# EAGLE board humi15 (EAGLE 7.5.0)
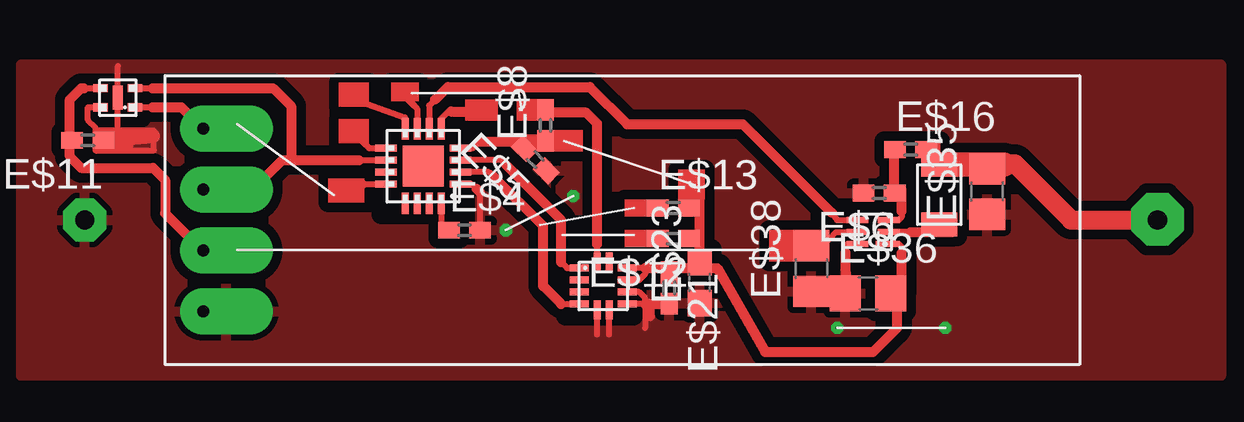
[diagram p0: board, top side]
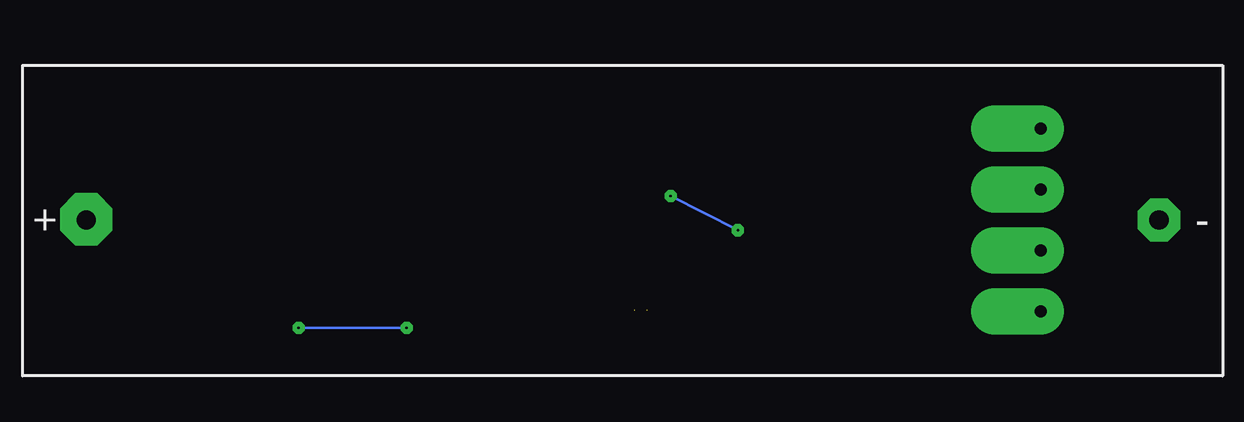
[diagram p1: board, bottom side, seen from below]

No outline drawn. Coordinates in mm, seen from the top.
Copper layers (1*16): Top 0.035mm / dielectric 1.5mm / Bottom 0.035mm
Design rules "default": minimum track width 10mil, minimum drill 24mil, track to track 8mil, track to pad 8mil, pad to pad 8mil, via to via 8mil, smd to smd 8mil, copper to edge 40mil, drill to drill 8mil, minimum pad ring 10mil, minimum via ring 8mil, stop-mask expansion 4mil, vias tented up to drill 0mil, thermal gap 10mil
tRestrict: area 22.7,2.5 to 25.5,5; area 15,6.7 to 18.5,10.5; area 3.1,10.8 to 5,12.2; area 34,4.8 to 36.9,7

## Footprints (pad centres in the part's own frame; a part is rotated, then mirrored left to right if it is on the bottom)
AAA_BATT = drill 0.8 pad 1.778 octagon: P$1 22.35,0; P$2 -22.35,0
OLED_128X32 = drill 0.5 pad 1.93 offset: 1 3.81,-1.587; 2 1.27,-1.587; 3 -1.27,-1.587; 4 -3.81,-1.587
QFN3X3_16 = smd 0.9 x 0.28: 1 -1.8,1; 2 -1.8,0.5; 3 -1.8,0; 4 -1.8,-0.5; 9 1.3,-0.5; 10 1.3,0; 11 1.3,0.5; 12 1.3,1 | smd 0.28 x 0.9: 5 -1,-1.3; 6 -0.5,-1.3; 7 0,-1.3; 8 0.5,-1.3; 13 0.5,1.8; 14 0,1.8; 15 -0.5,1.8; 16 -1,1.8 | smd 1.7 x 1.7: EP -0.25,0.25
C0402 = smd 0.9 x 0.7: 1 -0.65,0; 2 0.65,0
LGA12 = smd 0.8 x 0.3: 1 -0.75,0.5; 2 -0.75,0; 3 -0.75,-0.5; 4 -0.75,-1; 7 1.25,-1; 8 1.25,-0.5; 9 1.25,0; 10 1.25,0.5 | smd 0.3 x 0.8: 5 0,-1.25; 6 0.5,-1.25; 11 0.5,0.75; 12 0,0.75
DSE = smd 0.25 x 1: 1 -0.5,-0.6 | smd 0.25 x 0.9: 2 0,-0.65; 3 0.5,-0.65; 4 0.5,0.65; 5 0,0.65; 6 -0.5,0.65
SH4X = smd 0.6 x 0.35: 1 -0.725,0.4; 2 -0.725,-0.4; 3 0.725,-0.4; 4 0.725,0.4 | smd 0.4 x 1: EP 0,0
C0603 = smd 1.1 x 1: 1 -0.85,0; 2 0.85,0
C0805 = smd 1.3 x 1.5: 1 -0.95,0; 2 0.95,0
L1008 = smd 1 x 1.5: P$1 -1.25,0; P$2 1.25,0

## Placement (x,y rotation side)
E$1  [AAA_BATT]  25,6.5 180 bottom
E$2  [OLED_128X32]  6,6.5 90 top
E$3  [QFN3X3_16]  16.5,9 180 top
E$4  [C0402]  18.48,6.08 0 top
E$5  [C0402]  21.43,9.02 135 top
E$6  [C0402]  35.75,7.62 180 top
E$7  [LGA12]  24,4 0 top
E$8  [C0402]  21.85,10.45 90 top
E$9  [DSE]  35.5,6 90 top
E$10  [SH4X]  4.03,11.6 180 top
E$11  [C0402]  2.77,9.82 180 top
E$12  [C0402]  27.18,5.72 180 top
E$13  [C0402]  27.18,7 0 top
E$16  [C0402]  37.06,9.44 0 top
E$21  [C0402]  27,3.67 270 top
E$23  [C0603]  28.28,3.89 90 top
E$35  [C0805]  40.25,7.69 90 top
E$36  [C0805]  35.29,3.44 0 top
E$38  [C0805]  32.92,4.47 90 top
E$47  [L1008]  38.25,7.56 90 top

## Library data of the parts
E$1 = sb
E$2 = display-lcd
E$3 = renesas
E$4-E$6 E$8 E$11-E$13 E$16 E$21 E$23 E$35 E$36 E$38 = ref-packages
E$7 = st-microelectronics
E$9 = texas
E$10 = sensor
E$47 = rcl

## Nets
GND: E$1.P$2 E$2.4 E$4.2 E$5.1 E$6.2 E$7.5 E$7.6 E$11.1 E$21.2 E$23.1 E$35.1 E$36.1 E$38.1

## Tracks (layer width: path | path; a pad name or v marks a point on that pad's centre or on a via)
GND  (via drill 0.1 pad 0.3)  (2 unrouted)
  Top 0.254: 3.33,11.2 2.77,11.2 2.77,10.68 3.1,10.35 3.1,10.22 4.03,10.22 | 4.03,10.22 4.03,12.93 | 4.03,10.22 5.53,10.22 5.53,9.4 3.1,9.4 3.1,9.93 | 24.5,1.72 E$7.6 | 24,1.72 E$7.5 | 25.5,3.5 25.75,3.5 26,3.25 26,3 | 26,3 25.5,3 | 26,3 26,2 | 34.48,5.5 34.41,5.5 34.35,5.44 34.35,5.14 | 18.5,8 18.77,8 18.98,7.8 | E$4.2 19.12,7.65
  Top 0.406: 26.2,3 26,3 | 26.2,3 27,3 | 26.2,2.5 26.2,3 | 34.38,3.56 34.35,5.14 | 19.12,7.65 18.98,7.8
  Top 0.61: E$11.1 5.47,10 | 32.88,3.56 34.38,3.56 | 4.38,9.62 3.38,9.62
  Bottom 0.1: v34,2 v38.5,2 | v20.2,6.08 v23,7.5
  pour Top (isolate 0.406): 0,0 0,13 50,13 50,0
IRQ
  Top 0.254: 24,5 24,5.5
  Top 0.406: 22.05,10.97 23.55,10.97 24,10.53 24,5.5
PWR
  Top 0.254: 25.5,4 25.75,4 26,4.25 26,4.5 25.5,4.5
  Top 0.406: 36.5,3 36.5,2 35.5,1 31,1 29,4.5 26,4.5
S$1
  Top 0.406: 28.27,4.95 28.27,7.95
S$2
  Top 0.254: 14.2,8 15,8
  Top 0.406: 13.1,8 14.2,8
S$3
  Top 0.254: 17.5,7 17.5,6
S$4
  Top 0.254: 14.35,9.65 14.5,9.5 15,9.5
  Top 0.3: 14.35,9.65 14,10 13.47,10
S$5
  Top 0.254: 14.07,9 15,9
  Top 0.406: 14.07,9 10.88,9 9.38,7.5
S$6
  Top 0.254: 18.8,9.53 18.77,9.5 18.52,9.5
  Top 0.305: 18.8,9.53 19.07,9.78
  Top 0.406: 19.07,9.78 20.62,9.78
  Top 0.61: 20.62,9.78 21.8,9.78
S$7
  Top 0.254: 17.5,10.5 17.5,10.72 17.8,11.03 17.9,11.03 | 18.98,11.03 19.07,11.03
  Top 0.406: 17.9,11.03 18.98,11.03
S$9
  Top 0.254: 16,10.5 16,10.78 14.38,11.35
S$10
  Top 0.8: 47.38,6.5 43.75,6.5 41.4,8.85 40.95,8.85
S$11
  Top 0.254: 33.77,6.8 34,6.5 34.5,6.5 | 17,10.5 17,11.28 17.25,11.53
  Top 0.406: 33.77,6.8 30.07,10.5 25.25,10.5 23.7,12.05 17.77,12.05 17.25,11.53
S$12
  Top 0.254: 16.38,11.28 16.5,11.15 16.5,10.5
  Top 0.3: 16.38,11.28 15.95,11.7
S$13  (via drill 0.6 pad 2.18)
  other vias: 47.35,6.53
S$14
  Top 0.406: 31.5,5.5 33,5.5
S$16
  Top 0.254: 4.65,11.2 5.47,11.2
  Top 0.406: 5.47,11.2 6.67,11.2 7.38,10.47
S$17
  Top 0.254: 4.62,12 5.47,12 | 5.95,12 6.08,12
  Top 0.406: 5.47,12 5.95,12 | 6.08,12 10.5,12 11.25,11.25 11.25,9
S$22
  Top 0.254: 35,6 33.95,6 33.41,5.44
S$23
  Top 0.254: 36.38,5.5 36.56,5.5 36.69,5.38 36.69,5.11
  Top 0.406: 36.69,3.5 36.69,5.11
S$28
  Top 0.254: 37.06,6 36.5,6
  Top 0.406: 37.06,6 38.79,6
S$35
  Top 1.016: 38,8.81 40.94,8.81
S$57
  Top 0.254: 36.5,6.5 36.56,6.5 36.69,6.62 36.69,6.88
  Top 0.305: 36.69,7.76 36.38,7.75
  Top 0.406: 36.69,6.88 36.69,7.76 | 36.38,7.75 36.38,9.06
SCL
  Top 0.254: 20.23,8.78 20,9 18.5,9 | 23,4.5 22.75,4.5 22.5,4.75
  Top 0.406: 20.23,8.78 22.5,6.5 22.5,4.75
SDA
  Top 0.254: 19.7,8.3 19.5,8.5 18.5,8.5 | 22.5,3 23,3
  Top 0.406: 19.7,8.3 21.75,6.25 21.75,3.75 22.5,3
SUB
  Top 0.254: 2.62,12 3.12,12
  Top 0.406: 2.62,12 2.5,12 2.02,11.53 2.02,9.15 2.5,8.68 5.5,8.68 6,8.18 6,6.78 7,5.78
(copper drawn outside any net)
  shapes: Top area x12

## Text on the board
Document: SWDIO | SWCLK | RES | SDA | SCL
